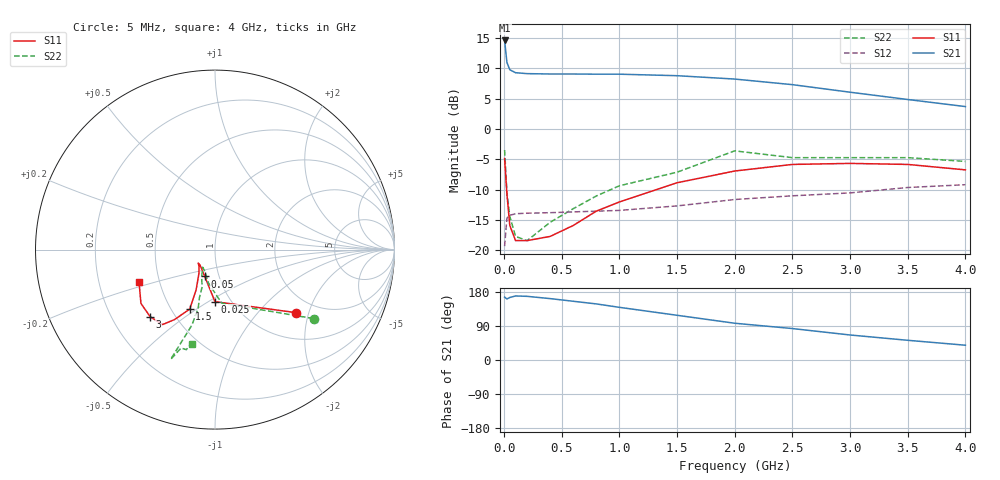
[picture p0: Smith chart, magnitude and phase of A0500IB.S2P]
!  MSA-0500 S PARAMETERS
!  Id=165mA  LAST UPDATED 07-22-92
# ghz s ma r 50
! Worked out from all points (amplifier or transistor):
!   15 points, 5 MHz to 4 GHz, reference 50 ohm
!   highest |S21| = 14.6 dB at 5 MHz (marker M1)
!   |S21| within 3 dB of that: start of sweep to 21.58 MHz
!   unconditionally stable (mu >= 1): 40.01 MHz to 757.7 MHz
!   at 50 MHz: K = 1.06, MAG = 10.5 dB, |S12| = -14.2 dB
!   at 800 MHz: K = 0.98, MSG = 11.3 dB, |S12| = -13.6 dB
!   at 4 GHz: K = 0.60, MSG = 6.4 dB, |S12| = -9.2 dB
!   S11 on the Smith chart (normalised r, x): 5 MHz: 1.58, -1.65; 25 MHz: 0.84, -0.54; 50 MHz: 0.85, -0.26; 1.5 GHz: 0.62, -0.47; 3 GHz: 0.37, -0.38; 4 GHz: 0.38, -0.17
0.005  0.57 -38.0  5.37 166.0  0.108 39.0  0.67 -35.0
0.025  0.29 -90.0  3.54 161.0  0.184 18.0  0.3 -83.0
0.05  0.16 -111.0  3.08 165.0  0.194 10.0  0.19 -101.0
0.1  0.12 -134.0  2.91 169.0  0.2 4.0  0.13 -117.0
0.2  0.12 -141.0  2.86 168.0  0.202 4.0  0.12 -125.0
0.4  0.13 -133.0  2.84 162.0  0.204 4.0  0.17 -116.0
0.6  0.16 -124.0  2.84 155.0  0.207 4.0  0.22 -109.0
0.8  0.21 -118.0  2.83 148.0  0.21 5.0  0.28 -108.0
1  0.25 -115.0  2.83 139.0  0.213 6.0  0.34 -106.0
1.5  0.36 -113.0  2.75 118.0  0.232 9.0  0.44 -107.0
2  0.45 -120.0  2.58 97.0  0.262 12.0  0.66 -112.0
2.5  0.51 -125.0  2.32 83.0  0.281 17.0  0.58 -109.0
3  0.52 -134.0  2.01 66.0  0.297 19.0  0.58 -109.0
3.5  0.51 -144.0  1.75 52.0  0.329 20.0  0.58 -106.0
4  0.46 -157.0  1.53 39.0  0.347 21.0  0.54 -104.0
